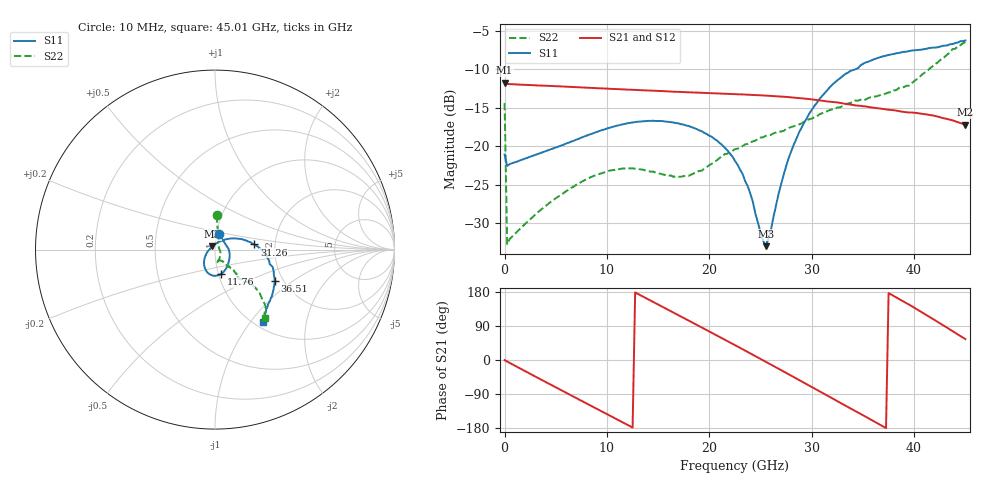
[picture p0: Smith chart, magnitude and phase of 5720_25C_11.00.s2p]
! Device:  ADRF5720
! Description: 0.5dB LSB GaAs MMIC 6-bit Digital Attenuator
! Frequency:  0.000009 -  40 GHz
! Ports:
!	RF1	= Port 1
!	RF2	= Port 2
! Vdd:  3.3 Volt
! Vss:  -3.3 Volt
! Control:  0/3.3 Volt
! State:  11.00 dB attenuation
! Data:  The device was measured using G-S-G Probes on a matrix board.
!  Data was collected using an calibrated 4 port network analyzer.
!  The reference plane for this measurement is at the launchers.
! Note:  Analog Devices supplies this data as a sample of measured data
!  for this product.  Your particular data for this product may vary.
!  Data was taken at 25 degrees C.
!  Analog Devices reserves the right to change this data at anytime.
# GHZ S DB R 45.0
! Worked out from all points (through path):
!   181 points, 10 MHz to 45.01 GHz, reference 45 ohm
!   highest |S21| = -11.74 dB at 10 MHz (marker M1); lowest = -17.2 dB at 45.01 GHz (marker M2)
!   group delay of S21, straight-line fit = 40.6 ps
!   lowest |S11| = -33.0 dB at 25.51 GHz (marker M3), VSWR 1.05, Z = 43.7 + j1.52 ohm
!   |S11| at or under -10 dB: start of sweep to 34.28 GHz
!   |S22| runs from -32.8 to -6.5 dB; largest |S21 - S12| = 0.00035
!   S11 on the Smith chart (normalised r, x): 10 MHz: 1.03, +0.18; 11.76 GHz: 1.03, -0.28; 31.26 GHz: 1.56, +0.09; 36.51 GHz: 1.80, -0.73; 45.01 GHz: 1.09, -1.16
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0.01  -21.10 75.5  -11.74 -0.5  -11.74 -0.5  -14.41 87.1
0.26  -22.57 4.9  -11.92 -4.0  -11.92 -4.0  -32.76 18.9
4.26  -20.54 -31.0  -12.16 -61.5  -12.17 -61.5  -27.52 -45.9
7.76  -18.76 -53.6  -12.38 -111.1  -12.38 -111.1  -24.47 -67.3
11.76  -17.11 -75.9  -12.64 -167.7  -12.64 -167.6  -22.91 -81.8
15.26  -16.73 -94.0  -12.83 142.7  -12.84 142.8  -23.60 -83.4
17.26  -17.16 -104.0  -12.96 114.4  -12.96 114.4  -23.98 -74.0
19.01  -17.95 -113.3  -13.05 89.4  -13.05 89.4  -23.23 -62.9
21.26  -19.86 -126.7  -13.18 57.2  -13.18 57.2  -21.28 -55.5
22.76  -22.42 -140.2  -13.26 35.6  -13.26 35.6  -20.33 -53.0
24.01  -26.19 -158.6  -13.34 17.4  -13.34 17.5  -19.49 -52.6
25.51  -33.01 129.2  -13.42 -4.5  -13.43 -4.4  -18.66 -52.5
27.76  -21.52 43.6  -13.63 -37.8  -13.64 -37.8  -17.64 -49.5
28.76  -18.24 30.8  -13.75 -52.7  -13.75 -52.6  -17.19 -49.0
30.26  -14.78 16.1  -13.96 -75.2  -13.97 -75.1  -16.23 -48.2
31.26  -13.10 7.5  -14.15 -90.1  -14.15 -90.0  -15.57 -48.5
33.26  -10.64 -7.9  -14.50 -119.9  -14.50 -119.9  -14.56 -48.8
36.51  -8.51 -27.7  -15.09 -168.3  -15.09 -168.2  -13.45 -50.4
37.76  -8.07 -34.3  -15.30 172.9  -15.30 173.0  -12.98 -47.9
39.51  -7.65 -41.7  -15.63 146.1  -15.63 146.2  -12.14 -46.4
41.76  -7.20 -48.5  -15.99 109.7  -15.99 109.8  -9.68 -43.9
45.01  -6.26 -56.6  -17.22 55.1  -17.22 55.2  -6.46 -53.7
